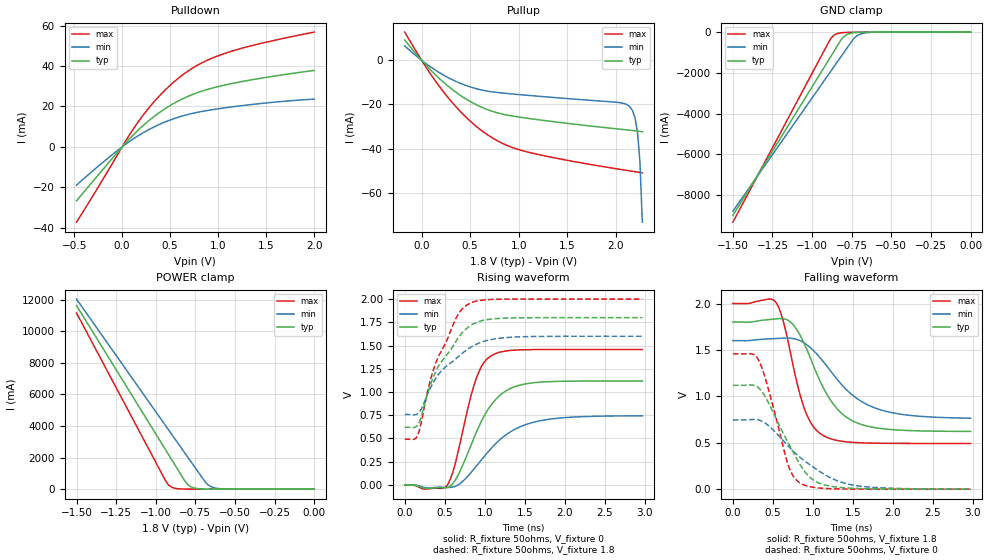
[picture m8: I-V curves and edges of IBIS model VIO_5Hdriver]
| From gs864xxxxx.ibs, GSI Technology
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|  signals   DQA1-DQA9, DQB1-DQB9, DQC1-DQC9, DQD1-DQD9
[Model]   VIO_5Hdriver
Model_type   I/O
Polarity   Non-Inverting
Vinl  =   0.75v
Vinh  =   1.75v
Vmeas =   0.9v
Cref  =   0pF
Rref  =   50
Vref  =   0.9v
|  variable   typ   min   max
C_comp   3.0pF   2.5pF   3.5pF
|  variable   typ   min   max
[Temperature Range]   50   0   100
|  variable   typ   min   max
[Voltage Range]   1.8   1.6   2.0
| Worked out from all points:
|   slope of the pulldown table from 0 to 0.27 V, typ, clamps not added: 21.3 ohm
|   slope of the pullup table from 0 to 0.27 V, typ, clamps not added: 23.3 ohm
|   GND clamp passes 1 mA (typ) near -0.58 V on its own axis
|   POWER clamp passes 1 mA (typ) near -0.61 V on its own axis
|   rising waveform, R_fixture 50ohms, V_fixture 0: 20-80 % time 381ps typ, 526ps min, 253ps max; typ from 0 V to 1.12 V
|   rising waveform, R_fixture 50ohms, V_fixture 1.8: 20-80 % time 409ps typ, 481ps min, 359ps max; typ from 0.621 V to 1.8 V
|   falling waveform, R_fixture 50ohms, V_fixture 1.8: 20-80 % time 418ps typ, 562ps min, 265ps max; typ from 1.8 V to 0.622 V
|   falling waveform, R_fixture 50ohms, V_fixture 0: 20-80 % time 405ps typ, 612ps min, 265ps max; typ from 1.12 V to 0 V
[Pulldown]
| voltage   typ   min   max
-475mV    -26.66mA   -18.97mA   -37.28mA
-75mV     -4.15mA    -2.792mA   -6.079mA
50mV      2.67mA     1.772mA    3.957mA
175mV     8.69mA     5.747mA    12.88mA
275mV     12.88mA    8.483mA    19.1mA
375mV     16.55mA    10.85mA    24.58mA
475mV     19.73mA    12.86mA    29.38mA
600mV     23.09mA    14.91mA    34.52mA
825mV     27.51mA    17.48mA    41.49mA
1.1V      30.94mA    19.53mA    46.76mA
1.45V     34.01mA    21.5mA     51.28mA
2V        37.83mA    23.65mA    56.83mA
[Pullup]
| voltage (VDDQ-Vout) typ   min   max
-175mV    9.211mA    6.502mA    12.78mA
75mV      -3.6mA     -2.462mA   -5.118mA
275mV     -11.79mA   -7.883mA   -17.04mA
500mV     -18.63mA   -12.05mA   -27.52mA
725mV     -23.05mA   -14.27mA   -35.04mA
1.1V      -26.3mA    -15.89mA   -41.6mA
2.125V    -31.57mA   -20.29mA   -49.93mA
2.175V    -31.8mA    -22.89mA   -50.27mA
2.2V      -31.92mA   -26.11mA   -50.44mA
2.225V    -32.05mA   -32.53mA   -50.6mA
2.25V     -32.19mA   -45.73mA   -50.77mA
2.275V    -32.35mA   -73.31mA   -50.94mA
[GND Clamp]
| voltage   typ   min   max
-1.5V     -9.007A    -8.796A    -9.334A
-900mV    -1.426A    -2.122A    -562.9mA
-880mV    -1.174A    -1.9A      -292.9mA
-860mV    -921.1mA   -1.678A    -142.5mA
-820mV    -416.2mA   -1.233A    -38.58mA
-800mV    -222mA     -1.011A    -23.51mA
-780mV    -116.3mA   -788.8mA   -16.2mA
-740mV    -33.04mA   -348.7mA   -9.876mA
-720mV    -18.57mA   -198.2mA   -8.142mA
-680mV    -6.87mA    -61.92mA   -5.539mA
-580mV    -1.002mA   -3.885mA   -1.438mA
0V        -402.5pA   -791.6pA   -356.8pA
[POWER Clamp]
| voltage (VDDQ-Vout) typ   min   max
-1.5V     11.62A     12.03A     11.14A
-940mV    2.526A     4.049A     574.2mA
-920mV    2.201A     3.764A     270.7mA
-900mV    1.877A     3.479A     123.3mA
-880mV    1.552A     3.194A     56.51mA
-820mV    578.6mA    2.34A      8.04mA
-800mV    303.9mA    2.055A     5.265mA
-760mV    77.74mA    1.486A     2.987mA
-680mV    5.757mA    367.3mA    1.268mA
-640mV    1.972mA    111.8mA    748.9uA
-540mV    239.3uA    5.502mA    108.9uA
0V        575.4pA    0A         0A
[Ramp]
| voltage   typ   min   max
dV/dt_r   1.53/137p   1.35/170p   1.77/112p
dV/dt_f   1.51/136p   1.31/167p   1.77/112p
R_load  =   50ohms
[Rising Waveform]
C_fixture =   0.0pf
R_fixture =   50ohms
V_fixture =   0
| Time   V(typ)   V(min)   V(max)
0s        5.368nV    14.01nV    3.516nV
270ps     -38.36mV   -30.53mV   -45.25mV
540ps     -26.5mV    -26.58mV   7.303mV
660ps     93.43mV    -3.531mV   329.2mV
810ps     388.6mV    114.7mV    896.5mV
900ps     576.3mV    207.1mV    1.161V
1.08ns    860.8mV    392.8mV    1.389V
1.32ns    1.038V     570.9mV    1.447V
1.68ns    1.105V     688.3mV    1.457V
2.97ns    1.119V     744.3mV    1.458V
[Rising Waveform]
C_fixture =   0.0pf
R_fixture =   50ohms
V_fixture =   1.8
V_fixture_min =   1.6
V_fixture_max =   2.0
| Time   V(typ)   V(min)   V(max)
0s        620.9mV    758.2mV    492.4mV
150ps     631.1mV    759.7mV    513.2mV
210ps     740.8mV    818.3mV    680.2mV
300ps     1.022V     1.005V     1.06V
390ps     1.224V     1.149V     1.316V
660ps     1.572V     1.373V     1.823V
780ps     1.688V     1.456V     1.938V
960ps     1.767V     1.536V     1.987V
1.32ns    1.797V     1.589V     1.999V
2.97ns    1.8V       1.6V       2V
[Falling Waveform]
C_fixture =   0.0pf
R_fixture =   50ohms
V_fixture =   1.8
V_fixture_min =   1.6
V_fixture_max =   2.0
| Time   V(typ)   V(min)   V(max)
0s        1.8V       1.6V       2V
540ps     1.834V     1.623V     2.011V
630ps     1.836V     1.627V     1.809V
720ps     1.801V     1.627V     1.468V
900ps     1.553V     1.57V      852.5mV
1.02ns    1.303V     1.482V     657.2mV
1.14ns    1.076V     1.363V     572.7mV
1.38ns    801mV      1.107V     513.9mV
1.77ns    663.7mV    877.2mV    495.5mV
2.97ns    622.2mV    764.7mV    492.6mV
[Falling Waveform]
C_fixture =   0.0pf
R_fixture =   50ohms
V_fixture =   0
| Time   V(typ)   V(min)   V(max)
0s        1.119V     745.4mV    1.458V
240ps     1.123V     750.5mV    1.458V
330ps     1.086V     744.1mV    1.377V
450ps     922.6mV    680.5mV    1.059V
690ps     502.9mV    466.9mV    261.7mV
750ps     406.6mV    413.2mV    146.9mV
840ps     263.8mV    341.9mV    66.09mV
1.08ns    64.41mV    193.6mV    12.37mV
1.5ns     9.562mV    44.5mV     918.7uV
2.97ns    34.17uV    726.2uV    703.5nV
